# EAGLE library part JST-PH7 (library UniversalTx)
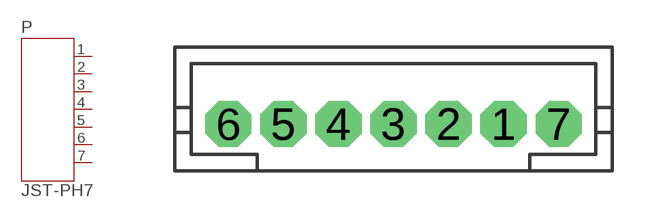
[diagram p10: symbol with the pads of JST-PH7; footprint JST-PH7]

Designator prefix P

## JST-PH7  [JST-PH7]
1  1  pas
2  2  pas
3  3  pas
4  4  pas
5  5  pas
6  6  pas
7  7  pas

## Footprint JST-PH7 (pad centres in mm)
drill 0.813 pad 1.676 octagon: 1 4,0; 2 2,0; 3 0,0; 4 -2,0; 5 -4,0; 6 -6,0; 7 6,0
